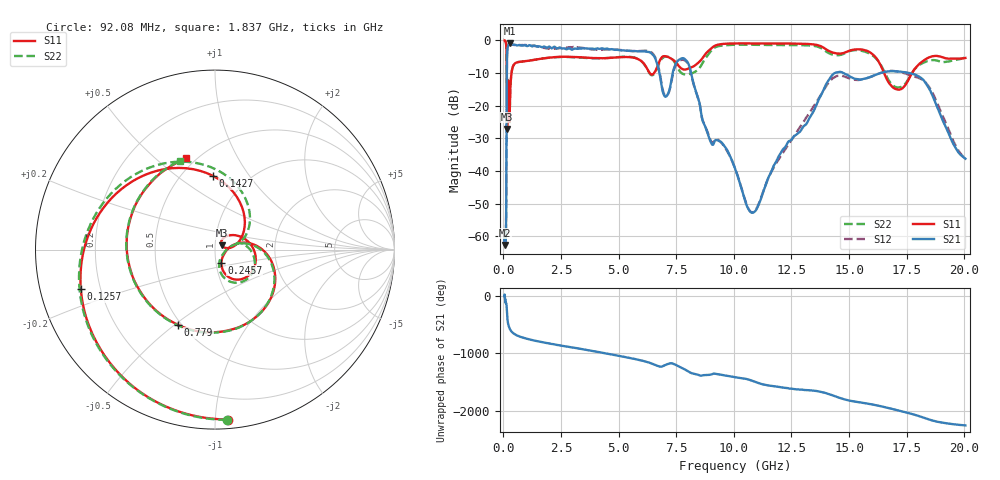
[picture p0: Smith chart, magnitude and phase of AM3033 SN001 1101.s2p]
# Hz S DB R 50
!freq MagS11 AngS11 MagS21 AngS21 MagS12 AngS12 MagS22 AngS22
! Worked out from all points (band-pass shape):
!   1601 points, 50 MHz to 20.05 GHz, reference 50 ohm
!   highest |S21| = -0.96 dB at 277 MHz (marker M1); lowest = -62.7 dB at 72.18 MHz (marker M2)
!   |S21| within 3 dB of the highest: 159.3 MHz to 6.408 GHz (6.248 GHz wide, 190 % of centre)
!   lowest |S11| = -27.2 dB at 159.7 MHz (marker M3), VSWR 1.09, Z = 53.8 + j2.54 ohm
!   |S11| at or under -10 dB: 145.5 MHz to 350.7 MHz (205.2 MHz wide, 82.7 % of centre); 6.343 GHz to 6.545 GHz (202.7 MHz wide, 3.15 % of centre); 16.52 GHz to 17.74 GHz (1.217 GHz wide, 7.11 % of centre)
!   |S22| runs from -25.9 to -0.1 dB; largest |S21 - S12| = 0.064
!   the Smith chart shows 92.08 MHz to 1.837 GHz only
!   S11 on the Smith chart (normalised r, x): 92.08 MHz: 0.06, -1.08; 125.7 MHz: 0.13, -0.14; 142.7 MHz: 0.70, +0.69; 245.7 MHz: 1.06, -0.15; 779 MHz: 0.48, -0.51; 1.837 GHz: 0.45, +0.63
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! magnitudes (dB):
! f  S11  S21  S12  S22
! 50 MHz  -0.1  -60.3  -58.6  -0.1
! 72.18 MHz  -0.2  -62.7  -61.7  -0.2
! 92.08 MHz  -0.4  -59.9  -60.0  -0.4
! 112.3 MHz  -1.1  -57.8  -57.2  -1.1
! 125.7 MHz  -2.2  -40.2  -40.2  -2.2
! 135.9 MHz  -4.3  -22.3  -22.3  -4.2
! 142.7 MHz  -7.7  -12.9  -12.9  -7.0
! 159.7 MHz  -27.2  -3.9  -3.9  -18.1
! 192.6 MHz  -12.5  -2.0  -2.0  -12.2
! 245.7 MHz  -21.9  -1.1  -1.1  -22.6
! 277 MHz  -19.8  -1.0  -1.0  -19.8
! 369.6 MHz  -9.2  -1.3  -1.2  -9.1
! 779 MHz  -6.6  -1.7  -1.6  -6.6
! 1.005 GHz  -6.4  -1.8  -1.5  -6.4
! 1.837 GHz  -5.5  -2.2  -2.4  -5.5
! 2.722 GHz  -5.1  -2.8  -2.4  -5.2
! 7.402 GHz  -6.2  -8.6  -9.1  -6.5
! 7.978 GHz  -8.8  -6.6  -6.9  -10.4
! 10.77 GHz  -1.0  -52.8  -52.6  -1.4
! 14.53 GHz  -4.1  -9.8  -10.9  -4.6
! 17.85 GHz  -8.8  -10.5  -11.2  -8.9
! 20.05 GHz  -5.5  -36.3  -36.1  -5.2
